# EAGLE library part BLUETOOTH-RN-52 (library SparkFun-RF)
Roving Networks RN-52 Bluetooth Audio Module The RN-52 is an audio module that provides a highly integrated solution for delivering high quality stereo audio in a small form factor with little difficulty. This module is perfect for a project involving hands free audio for your car, remote controlling your media center, or streaming 2-channel audio. SparkFun Products: RN-52 - Bluetooth Audio Module (WRL-11678) Audio Bluetooth Breakout - RN-52 (WRL-12849)
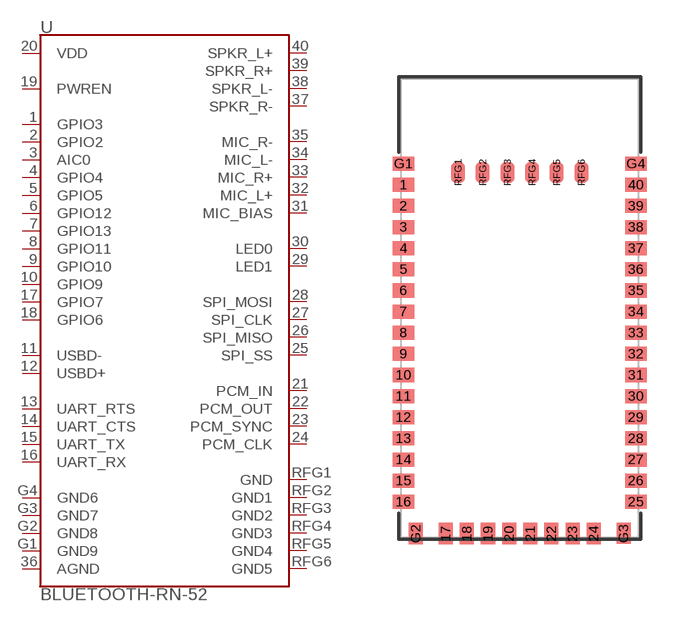
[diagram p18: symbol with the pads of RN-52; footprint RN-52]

Designator prefix -

## BLUETOOTH-RN-52 (PROD_ID: IC-11569; SF_ID: WRL-11678)  [RN-52]
1  GPIO3
2  GPIO2
3  AIC0
4  GPIO4
5  GPIO5
6  GPIO12
7  GPIO13
8  GPIO11
9  GPIO10
10  GPIO9
11  USBD-
12  USBD+
13  UART_RTS
14  UART_CTS
15  UART_TX
16  UART_RX
17  GPIO7
18  GPIO6
19  PWREN
20  VDD
21  PCM_IN
22  PCM_OUT
23  PCM_SYNC
24  PCM_CLK
25  SPI_SS
26  SPI_MISO
27  SPI_CLK
28  SPI_MOSI
29  LED1
30  LED0
31  MIC_BIAS
32  MIC_L+
33  MIC_R+
34  MIC_L-
35  MIC_R-
36  AGND
37  SPKR_R-
38  SPKR_L-
39  SPKR_R+
40  SPKR_L+
G1  GND9
G2  GND8
G3  GND7
G4  GND6
RFG1  GND
RFG2  GND1
RFG3  GND2
RFG4  GND3
RFG5  GND4
RFG6  GND5

## Footprint RN-52 (pad centres in mm)
Roving Networks RN-52 Bluetooth Audio Module 13.5x26.0x2.7mm module Datasheet
smd 1.2 x 0.8: 1 -6.6,8.33; 2 -6.6,7.13; 3 -6.6,5.93; 4 -6.6,4.73; 5 -6.6,3.53; 6 -6.6,2.33; 7 -6.6,1.13; 8 -6.6,-0.07; 9 -6.6,-1.27; 10 -6.6,-2.47; 11 -6.6,-3.67; 12 -6.6,-4.87; 13 -6.6,-6.07; 14 -6.6,-7.27; 15 -6.6,-8.47; 16 -6.6,-9.67; 25 6.6,-9.67; 26 6.6,-8.47; 27 6.6,-7.27; 28 6.6,-6.07; 29 6.6,-4.87; 30 6.6,-3.67; 31 6.6,-2.47; 32 6.6,-1.27; 33 6.6,-0.07; 34 6.6,1.13; 35 6.6,2.33; 36 6.6,3.53; 37 6.6,4.73; 38 6.6,5.93; 39 6.6,7.13; 40 6.6,8.33; G1 -6.6,9.53; G4 6.6,9.53
smd 0.8 x 1.2: 17 -4.2,-11.47; 18 -3,-11.47; 19 -1.8,-11.47; 20 -0.6,-11.47; 21 0.6,-11.47; 22 1.8,-11.47; 23 3,-11.47; 24 4.2,-11.47; G2 -5.9,-11.47; G3 5.9,-11.46; RFG1 -3.5,9.03; RFG2 -2.1,9.03; RFG3 -0.7,9.03; RFG4 0.7,9.03; RFG5 2.1,9.03; RFG6 3.5,9.03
